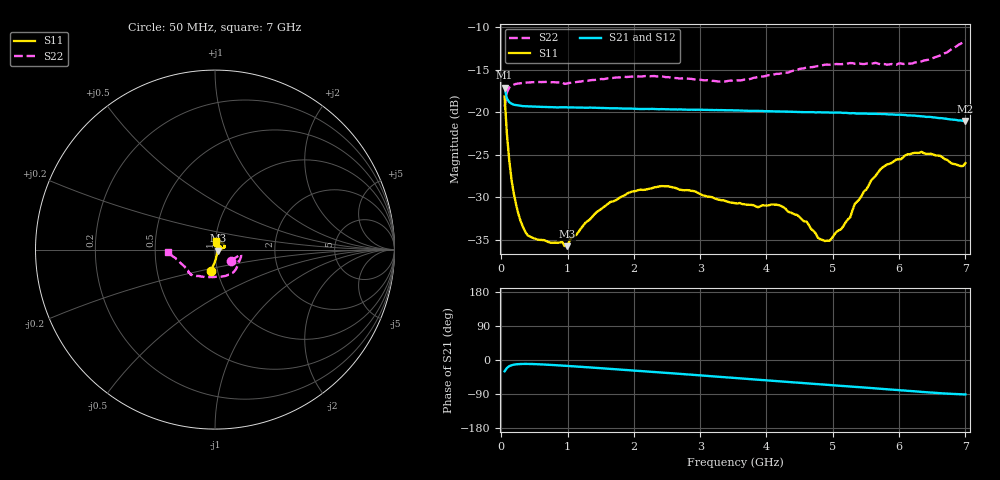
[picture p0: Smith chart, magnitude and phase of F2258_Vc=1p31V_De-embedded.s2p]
! Integrated Device Technology
! Corporate Headquarters
! 6024 Silver Creek Valley Road
! San Jose, CA 95138  USA
! Phone:  1-408-284-8200
! Toll Free:  1-800-223-1366
! Webpage:  http://www.idt.com/
! Timing and RF Division
! 515 Groton Road, Suite 102
! Westford, MA 01886-6024
! Device:  F2258
! Description: Voltage Variable RF Attenuator
! Frequency:  50.0 -  6000.00 MHz
! Package:  3x3 mm Thin QFN Plastic Package: 16 pin
! Ports:  2 RF, 2 DC
!  Pin  1  = NC
!  Pin  2  = NC
!  Pin  3  = RF2  = Port 2
!  Pin  4  = GND
!  Pin  5  = Vdd
!  Pin  6  = NC
!  Pin  7  = VCTRL
!  Pin  8  = NC
!  Pin  9  = GND
!  Pin 10  = RF1  = Port 1
!  Pin 11  = NC
!  Pin 12  = NC
!  Pin 13  = NC
!  Pin 14  = NC
!  Pin 15  = NC
!  Pin 16  = NC
! Vcntrl:  1.310 Volts
! Vdd:  +3.300 Volts
! Current:  1.167 mA
! Data:  The device was measured on a the F2258 evaluation board which has
!  individual transmission lines to the RF pins.  Data was collected
!  using a calibrated network analyzer.  The evaluation board was
!  de-embedded using a TRL calibration technique.
!  The reference plane is the edge of the package pin.
! Misc:  SN 10
!  Action Tracker AT0285
! Date Measured:  2014-12-10
! Date:  2016-01-13  MJV
! Note:
!  Integrated Device Technology supplies this data as a sample of measured
!  data at the package pin for this product.  Your particular data for this
!  product may vary.
!  Data was taken at 25 degrees C.
!  Integrated Device Technology reserves the right to change this data at anytime.
!Freq_(GHz)  S11M_(dB)  S11P_(deg)  S21M_(dB)  S21P_(deg)  S12M_(dB)  S12P_(deg)  S22M_(dB)  S22P_(deg)
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# GHz S dB R 50
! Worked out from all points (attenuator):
!   201 points, 50 MHz to 7 GHz, reference 50 ohm
!   highest |S21| = -17.10 dB at 50 MHz (marker M1); lowest = -21.0 dB at 7 GHz (marker M2)
!   lowest |S11| = -35.7 dB at 988.2 MHz (marker M3), VSWR 1.03, Z = 51.5 - j0.607 ohm
!   |S11| at or under -10 dB: start of sweep to end of sweep
!   |S22| runs from -19.4 to -11.6 dB; largest |S21 - S12| = 0.0007
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0.05  -18.15 -101.6  -17.10 -29.9  -17.11 -29.9  -19.37 -34.7
0.08475  -22.56 -92.4  -18.39 -21.0  -18.39 -21.0  -17.66 -16.7
0.15425  -27.92 -79.6  -18.99 -13.8  -19.01 -13.8  -16.87 -11.2
0.22375  -30.88 -69.2  -19.17 -11.4  -19.18 -11.4  -16.67 -10.3
0.328  -33.51 -53.6  -19.28 -10.4  -19.29 -10.4  -16.55 -11.7
0.467  -34.75 -38.6  -19.34 -10.6  -19.32 -10.6  -16.47 -14.0
0.98825  -35.75 -21.1  -19.42 -15.5  -19.43 -15.4  -16.63 -26.8
1.2315  -33.37 -9.9  -19.46 -18.3  -19.48 -18.3  -16.34 -32.3
1.6485  -30.53 -1.1  -19.53 -23.5  -19.56 -23.4  -16.01 -41.3
2.37825  -28.73 17.2  -19.65 -32.5  -19.66 -32.5  -15.78 -57.1
3.525  -30.71 70.2  -19.79 -47.5  -19.82 -47.4  -16.30 -94.4
4.22  -31.02 98.4  -19.92 -56.6  -19.92 -56.6  -15.43 -118.3
4.7065  -33.94 84.0  -19.99 -62.8  -20.00 -62.8  -14.68 -128.0
4.776  -34.75 78.6  -20.01 -63.8  -20.03 -63.7  -14.57 -129.0
4.94975  -35.12 55.0  -20.04 -66.0  -20.08 -65.9  -14.41 -131.0
5.2625  -32.36 22.1  -20.12 -69.9  -20.13 -69.9  -14.21 -134.6
5.332  -30.77 18.0  -20.12 -70.9  -20.12 -70.9  -14.31 -135.0
5.57525  -28.06 11.4  -20.18 -73.9  -20.19 -73.9  -14.31 -138.4
5.85325  -26.07 11.8  -20.26 -77.6  -20.26 -77.6  -14.37 -142.8
6.33975  -24.66 21.7  -20.48 -84.2  -20.50 -84.2  -14.02 -154.9
6.9305  -26.33 73.1  -20.97 -90.4  -21.03 -90.2  -11.94 -174.2
7  -25.98 83.9  -21.04 -90.8  -21.07 -90.7  -11.56 -176.8
